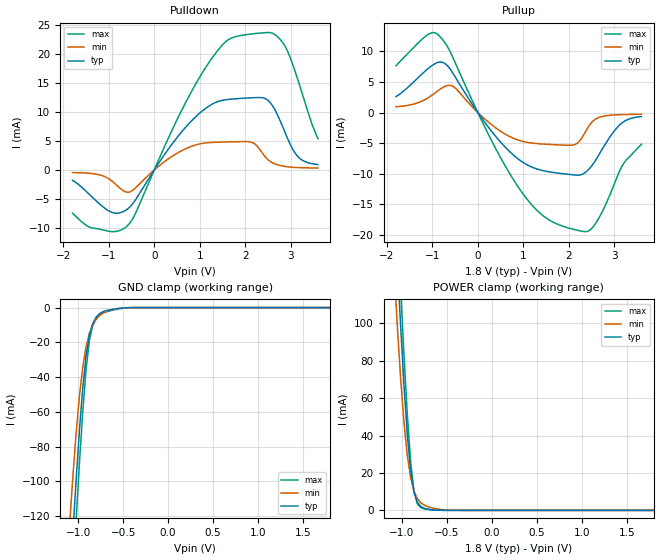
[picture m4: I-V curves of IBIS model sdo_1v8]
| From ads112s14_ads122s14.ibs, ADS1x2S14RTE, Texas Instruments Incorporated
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|   Model sdo_1v8
[Model] sdo_1v8
Model_type 3-state
Polarity   Non-Inverting
Enable   Active-High
C_comp   1.600pF   0.800pF   3.200pF
[Temperature Range]   27.000   0.125k   -40.000
[Voltage Range]   1.800V   1.650V   1.950V
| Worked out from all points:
|   slope of the pulldown table from 0 to 0.27 V, typ, clamps not added: 85.7 ohm
|   slope of the pullup table from 0 to 0.27 V, typ, clamps not added: 97.9 ohm
|   GND clamp passes 1 mA (typ) near -0.62 V on its own axis
|   POWER clamp passes 1 mA (typ) near -0.74 V on its own axis
[Pulldown]
|Voltage   I(typ)   I(min)   I(max)
-1.8V     -1.779mA   -445.5uA   -7.424mA
-1.415V   -4.303mA   -575.6uA   -9.871mA
-975mV    -7.154mA   -1.642mA   -10.58mA
-590mV    -6.736mA   -3.848mA   -9.606mA
840mV     8.618mA    4.133mA    13.8mA
1.39V     11.77mA    4.782mA    20.52mA
1.775V    12.25mA    4.861mA    22.94mA
2.16V     12.43mA    4.729mA    23.44mA
2.435V    12.32mA    2.325mA    23.64mA
2.82V     7.543mA    686.8uA    22.01mA
3.15V     2.387mA    413.8uA    15.74mA
3.6V      935uA      331.6uA    5.391mA
[Pullup]
|Voltage   I(typ)   I(min)   I(max)
-1.8V     2.598mA    947.9uA    7.66mA
-1.13V    6.961mA    2.243mA    12.59mA
-855mV    8.237mA    3.677mA    12.61mA
-525mV    6.154mA    4.178mA    8.603mA
245mV     -2.515mA   -1.646mA   -3.748mA
850mV     -7.378mA   -4.411mA   -11.75mA
1.345V    -9.336mA   -5.111mA   -16.31mA
1.895V    -10.04mA   -5.337mA   -18.66mA
2.17V     -10.24mA   -5.121mA   -19.23mA
2.5V      -8.774mA   -1.644mA   -19.01mA
3.105V    -2.136mA   -361.7uA   -9.798mA
3.6V      -660.7uA   -280.7uA   -5.188mA
[GND_clamp]
|Voltage   I(typ)   I(min)   I(max)
-1.8V     -906.9mA   -836.6mA   -952.9mA
-1.097V   -165.1mA   -126.9mA   -194.1mA
-1.06V    -131.4mA   -98.21mA   -157.8mA
-1.023V   -99.65mA   -72.66mA   -122.8mA
-986mV    -70.87mA   -51.1mA    -89.77mA
-949mV    -46.4mA    -34.34mA   -60.03mA
-912mV    -27.77mA   -22.5mA    -35.52mA
-875mV    -15.77mA   -14.85mA   -18.82mA
-838mV    -9.16mA    -10.03mA   -10.16mA
-764mV    -3.557mA   -4.737mA   -4.173mA
-431mV    -56.83uA   -62.45uA   -67.68uA
1.8V      0A         0A         0A
[POWER_clamp]
|Voltage   I(typ)   I(min)   I(max)
-1.8V     957.9mA    899.5mA    993.1mA
-1.086V   170mA      130.8mA    195.3mA
-1.049V   133.3mA    98.81mA    156.6mA
-1.012V   98.55mA    70.47mA    119mA
-975mV    66.97mA    46.97mA    83.44mA
-938mV    40.49mA    29.36mA    51.44mA
-901mV    21.29mA    17.57mA    25.92mA
-864mV    9.938mA    10.42mA    10.21mA
-827mV    4.429mA    6.356mA    3.552mA
-790mV    2.115mA    4.139mA    1.502mA
-457mV    2.391uA    60.32uA    338.6nA
1.8V      0A         0A         0A
[Ramp]
| variable   typ   min   max
dV/dt_r   0.986/0.604n   0.863/1.282n   1.099/0.328n
dV/dt_f   0.997/0.541n   0.855/1.334n   1.109/0.291n
R_load = 1.000k
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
